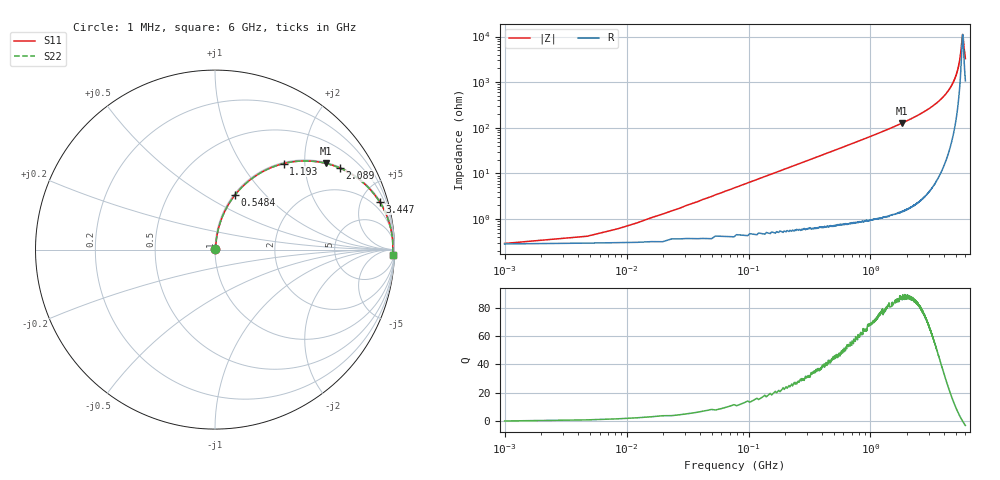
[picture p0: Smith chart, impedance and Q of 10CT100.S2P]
# MHZ S MA R 50
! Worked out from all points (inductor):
!   1601 points, 1 MHz to 6 GHz, reference 50 ohm
!   read as one part in series: L = 10 nH near 31 MHz
!   highest Q = 88 at 1.823 GHz (marker M1), where L = 11.1 nH
!   self-resonance near 5.701 GHz
!   S11 on the Smith chart (normalised r, x): 1 MHz: 1.01, +0.00; 548.4 MHz: 1.02, +0.69; 1.193 GHz: 1.02, +1.57; 2.089 GHz: 1.04, +3.03; 3.447 GHz: 1.12, +6.83; 6 GHz: 22, -63
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1  0.00277 13.0  0.997 -0.0  0.997 -0.0  0.00277 13.0
38.494  0.024 79.8  0.996 -1.4  0.996 -1.4  0.024 79.8
53.491  0.034 81.3  0.995 -1.9  0.995 -1.9  0.034 81.3
83.486  0.052 82.2  0.994 -3.0  0.994 -3.0  0.052 82.2
132.228  0.083 81.9  0.992 -4.7  0.992 -4.7  0.083 81.9
293.451  0.181 77.7  0.978 -10.4  0.978 -10.4  0.181 77.7
548.409  0.326 69.7  0.938 -19.0  0.938 -19.0  0.326 69.7
1002.083  0.541 56.4  0.833 -32.8  0.833 -32.8  0.541 56.4
1193.301  0.613 51.4  0.782 -37.8  0.782 -37.8  0.613 51.4
1823.196  0.783 37.8  0.613 -51.5  0.613 -51.5  0.783 37.8
2003.166  0.816 34.6  0.568 -54.7  0.568 -54.7  0.816 34.6
2089.402  0.83 33.2  0.548 -56.1  0.548 -56.1  0.83 33.2
3000.5  0.929 20.9  0.356 -68.3  0.356 -68.3  0.929 20.9
3446.676  0.955 16.2  0.28 -72.7  0.28 -72.7  0.955 16.2
4001.583  0.975 11.3  0.197 -77.0  0.197 -77.0  0.975 11.3
4590.235  0.986 6.9  0.12 -79.9  0.12 -79.9  0.986 6.9
5002.666  0.99 4.2  0.073 -80.0  0.073 -80.0  0.99 4.2
5385.103  0.991 1.8  0.033 -73.6  0.033 -73.6  0.991 1.8
5688.802  0.991 0.1  0.008974 -7.4  0.008974 -7.4  0.991 0.1
5741.293  0.991 -0.2  0.009833 23.2  0.009833 23.2  0.991 -0.2
5887.519  0.99 -1.0  0.02 61.2  0.02 61.2  0.99 -1.0
6000  0.99 -1.6  0.03 69.5  0.03 69.5  0.99 -1.6
